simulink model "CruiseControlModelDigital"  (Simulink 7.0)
settings: Solver=ode45  StartTime=0.0  StopTime=100  MaxStep=0.01  RelTol=1e-3
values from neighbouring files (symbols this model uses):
  g = 9.81    [CruiseControlDigital.m]
  m = 1000    [CruiseControlDigital.m]
libraries: cstblocks x10

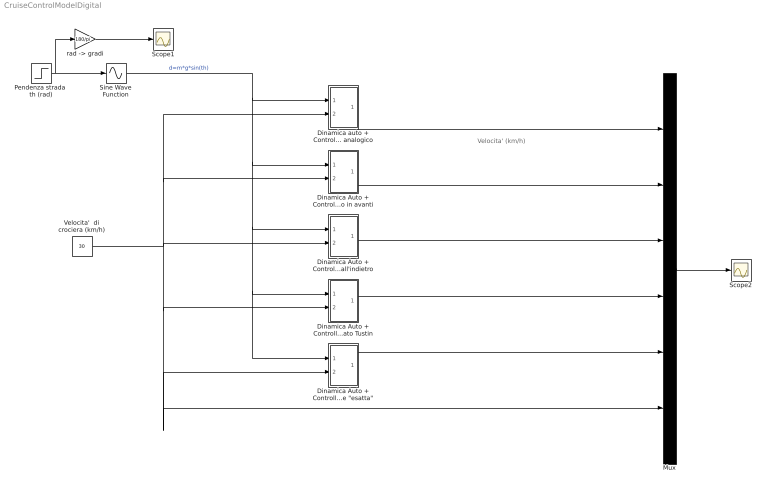
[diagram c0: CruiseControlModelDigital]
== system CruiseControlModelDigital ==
  note: Velocita' (km/h)
  "Dinamica Auto + Controllore digitalizzato Discretizzazione \"esatta\"" : Subsystem
  Dinamica Auto + Controllore digitalizzato Eulero all'indietro : Subsystem
  Dinamica Auto + Controllore digitalizzato Eulero in avanti : Subsystem
  Dinamica Auto + Controllore digitalizzato Tustin : Subsystem
  Dinamica auto + Controllore analogico : Subsystem
  Mux : Mux  Inputs=6
  Pendenza strada  th (rad) : Step  Time=20  After=5*pi/180  SampleTime=0
  Scope1 : Scope
  Scope2 : Scope
  Sine Wave Function : Sin  TimeSource=Use external signal  Amplitude=m*g  SampleTime=0
  Velocita'  di crociera (km/h) : Constant  Value=30  OutDataType=sfix(16)  OutScaling=2^0
  "rad -> gradi" : Gain  Gain=180/pi  ParameterDataType=sfix(16)  ParameterScaling=2^0  OutDataType=sfix(16)  OutScaling=2^0
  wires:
  Pendenza strada  th (rad)/1 -> Sine Wave Function/1, "rad -> gradi"/1
  "rad -> gradi"/1 -> Scope1/1
  Sine Wave Function/1 -> Dinamica auto + Controllore analogico/1(In1), Dinamica Auto + Controllore digitalizzato Eulero in avanti/1(In1), Dinamica Auto + Controllore digitalizzato Eulero all'indietro/1(In1), Dinamica Auto + Controllore digitalizzato Tustin/1(In1), "Dinamica Auto + Controllore digitalizzato Discretizzazione \"esatta\""/1(In1)  "d=m*g*sin(th)"
  Dinamica auto + Controllore analogico/1(Out1) -> Mux/1
  Dinamica Auto + Controllore digitalizzato Eulero in avanti/1(Out1) -> Mux/2
  Dinamica Auto + Controllore digitalizzato Eulero all'indietro/1(Out1) -> Mux/3
  Dinamica Auto + Controllore digitalizzato Tustin/1(Out1) -> Mux/4
  Mux/1 -> Scope2/1
  "Dinamica Auto + Controllore digitalizzato Discretizzazione \"esatta\""/1(Out1) -> Mux/5
  Velocita'  di crociera (km/h)/1 -> Dinamica Auto + Controllore digitalizzato Tustin/2(In2), "Dinamica Auto + Controllore digitalizzato Discretizzazione \"esatta\""/2(In2), Mux/6, Dinamica auto + Controllore analogico/2(In2), Dinamica Auto + Controllore digitalizzato Eulero in avanti/2(In2), Dinamica Auto + Controllore digitalizzato Eulero all'indietro/2(In2)

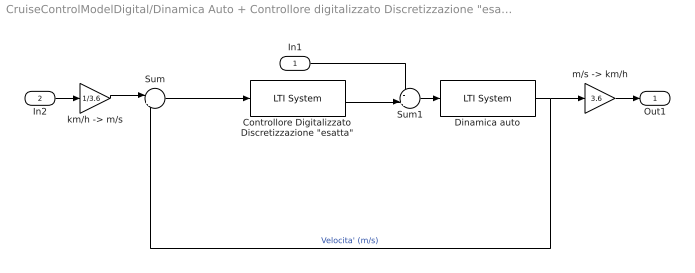
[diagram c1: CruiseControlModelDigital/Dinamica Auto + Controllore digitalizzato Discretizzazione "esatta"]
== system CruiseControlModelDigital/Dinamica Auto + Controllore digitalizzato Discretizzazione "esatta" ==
  In1 : Inport  OutDataType=sfix(16)  OutScaling=2^0
  In2 : Inport  Port=2  OutDataType=sfix(16)  OutScaling=2^0
  "Controllore Digitalizzato Discretizzazione \"esatta\"" : cstblocks/LTI System  SystemSampleTime=-1  sys=Cdz  IC=[]
  Dinamica auto : cstblocks/LTI System  SystemSampleTime=-1  sys=G  IC=[]
  Sum : Sum  Inputs=|+-  OutDataType=sfix(16)  OutScaling=2^0
  Sum1 : Sum  Inputs=-+|  OutDataType=sfix(16)  OutScaling=2^0
  "km/h -> m/s" : Gain  Gain=1/3.6  ParameterDataType=sfix(16)  ParameterScaling=2^0  OutDataType=sfix(16)  OutScaling=2^0
  "m/s -> km/h" : Gain  Gain=3.6  ParameterDataType=sfix(16)  ParameterScaling=2^0  OutDataType=sfix(16)  OutScaling=2^0
  Out1 : Outport  OutDataType=sfix(16)  OutScaling=2^0
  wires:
  "km/h -> m/s"/1 -> Sum/1
  "Controllore Digitalizzato Discretizzazione \"esatta\""/1 -> Sum1/2
  Sum1/1 -> Dinamica auto/1
  Dinamica auto/1 -> "m/s -> km/h"/1, Sum/2  "Velocita' (m/s)"
  Sum/1 -> "Controllore Digitalizzato Discretizzazione \"esatta\""/1
  In1/1 -> Sum1/1
  In2/1 -> "km/h -> m/s"/1
  "m/s -> km/h"/1 -> Out1/1

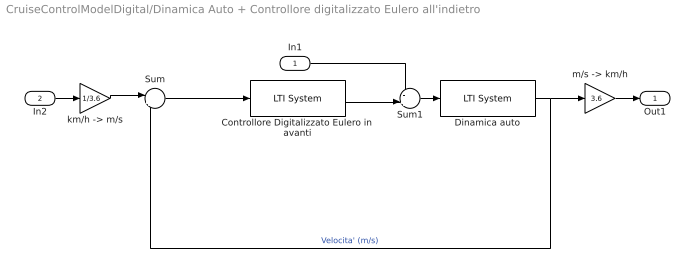
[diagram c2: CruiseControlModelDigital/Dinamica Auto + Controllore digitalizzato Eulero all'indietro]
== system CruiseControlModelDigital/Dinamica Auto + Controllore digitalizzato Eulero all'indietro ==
  In1 : Inport  OutDataType=sfix(16)  OutScaling=2^0
  In2 : Inport  Port=2  OutDataType=sfix(16)  OutScaling=2^0
  Controllore Digitalizzato Eulero in avanti : cstblocks/LTI System  SystemSampleTime=-1  sys=Cdb  IC=[]
  Dinamica auto : cstblocks/LTI System  SystemSampleTime=-1  sys=G  IC=[]
  Sum : Sum  Inputs=|+-  OutDataType=sfix(16)  OutScaling=2^0
  Sum1 : Sum  Inputs=-+|  OutDataType=sfix(16)  OutScaling=2^0
  "km/h -> m/s" : Gain  Gain=1/3.6  ParameterDataType=sfix(16)  ParameterScaling=2^0  OutDataType=sfix(16)  OutScaling=2^0
  "m/s -> km/h" : Gain  Gain=3.6  ParameterDataType=sfix(16)  ParameterScaling=2^0  OutDataType=sfix(16)  OutScaling=2^0
  Out1 : Outport  OutDataType=sfix(16)  OutScaling=2^0
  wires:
  "km/h -> m/s"/1 -> Sum/1
  Controllore Digitalizzato Eulero in avanti/1 -> Sum1/2
  Sum1/1 -> Dinamica auto/1
  Dinamica auto/1 -> "m/s -> km/h"/1, Sum/2  "Velocita' (m/s)"
  Sum/1 -> Controllore Digitalizzato Eulero in avanti/1
  In1/1 -> Sum1/1
  In2/1 -> "km/h -> m/s"/1
  "m/s -> km/h"/1 -> Out1/1

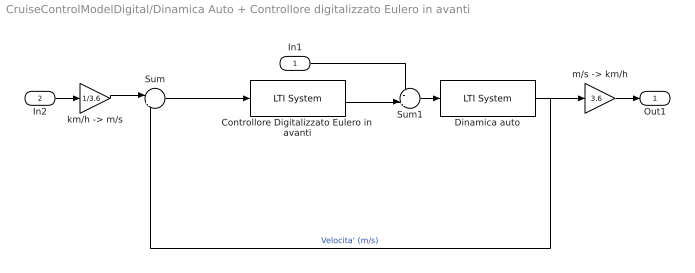
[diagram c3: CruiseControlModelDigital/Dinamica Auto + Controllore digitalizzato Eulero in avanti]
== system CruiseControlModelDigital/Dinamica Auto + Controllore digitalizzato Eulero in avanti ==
  In1 : Inport  OutDataType=sfix(16)  OutScaling=2^0
  In2 : Inport  Port=2  OutDataType=sfix(16)  OutScaling=2^0
  Controllore Digitalizzato Eulero in avanti : cstblocks/LTI System  SystemSampleTime=-1  sys=Cdf  IC=[]
  Dinamica auto : cstblocks/LTI System  SystemSampleTime=-1  sys=G  IC=[]
  Sum : Sum  Inputs=|+-  OutDataType=sfix(16)  OutScaling=2^0
  Sum1 : Sum  Inputs=-+|  OutDataType=sfix(16)  OutScaling=2^0
  "km/h -> m/s" : Gain  Gain=1/3.6  ParameterDataType=sfix(16)  ParameterScaling=2^0  OutDataType=sfix(16)  OutScaling=2^0
  "m/s -> km/h" : Gain  Gain=3.6  ParameterDataType=sfix(16)  ParameterScaling=2^0  OutDataType=sfix(16)  OutScaling=2^0
  Out1 : Outport  OutDataType=sfix(16)  OutScaling=2^0
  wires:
  "km/h -> m/s"/1 -> Sum/1
  Controllore Digitalizzato Eulero in avanti/1 -> Sum1/2
  Sum1/1 -> Dinamica auto/1
  Dinamica auto/1 -> "m/s -> km/h"/1, Sum/2  "Velocita' (m/s)"
  Sum/1 -> Controllore Digitalizzato Eulero in avanti/1
  In1/1 -> Sum1/1
  In2/1 -> "km/h -> m/s"/1
  "m/s -> km/h"/1 -> Out1/1

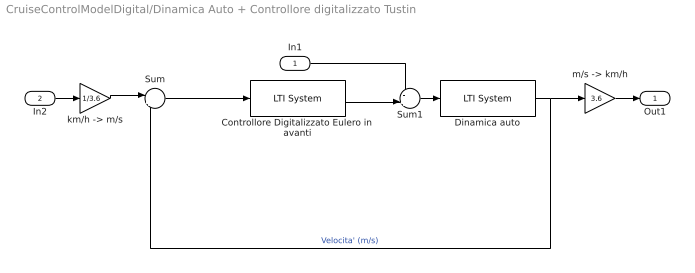
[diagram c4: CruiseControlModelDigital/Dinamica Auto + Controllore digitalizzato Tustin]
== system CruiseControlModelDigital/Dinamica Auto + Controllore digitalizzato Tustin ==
  In1 : Inport  OutDataType=sfix(16)  OutScaling=2^0
  In2 : Inport  Port=2  OutDataType=sfix(16)  OutScaling=2^0
  Controllore Digitalizzato Eulero in avanti : cstblocks/LTI System  SystemSampleTime=-1  sys=Cdt  IC=[]
  Dinamica auto : cstblocks/LTI System  SystemSampleTime=-1  sys=G  IC=[]
  Sum : Sum  Inputs=|+-  OutDataType=sfix(16)  OutScaling=2^0
  Sum1 : Sum  Inputs=-+|  OutDataType=sfix(16)  OutScaling=2^0
  "km/h -> m/s" : Gain  Gain=1/3.6  ParameterDataType=sfix(16)  ParameterScaling=2^0  OutDataType=sfix(16)  OutScaling=2^0
  "m/s -> km/h" : Gain  Gain=3.6  ParameterDataType=sfix(16)  ParameterScaling=2^0  OutDataType=sfix(16)  OutScaling=2^0
  Out1 : Outport  OutDataType=sfix(16)  OutScaling=2^0
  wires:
  "km/h -> m/s"/1 -> Sum/1
  Controllore Digitalizzato Eulero in avanti/1 -> Sum1/2
  Sum1/1 -> Dinamica auto/1
  Dinamica auto/1 -> "m/s -> km/h"/1, Sum/2  "Velocita' (m/s)"
  Sum/1 -> Controllore Digitalizzato Eulero in avanti/1
  In1/1 -> Sum1/1
  In2/1 -> "km/h -> m/s"/1
  "m/s -> km/h"/1 -> Out1/1

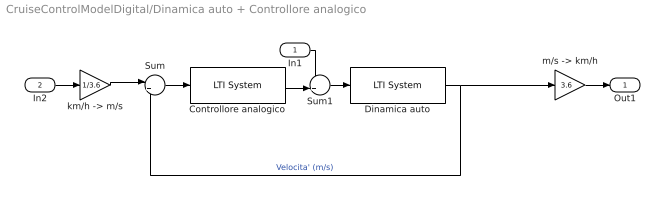
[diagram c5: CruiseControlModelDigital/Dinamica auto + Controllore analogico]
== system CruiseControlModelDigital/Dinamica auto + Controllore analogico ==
  In1 : Inport  OutDataType=sfix(16)  OutScaling=2^0
  In2 : Inport  Port=2  OutDataType=sfix(16)  OutScaling=2^0
  Controllore analogico : cstblocks/LTI System  SystemSampleTime=-1  sys=C  IC=[]
  Dinamica auto : cstblocks/LTI System  SystemSampleTime=-1  sys=G  IC=[]
  Sum : Sum  Inputs=|+-  OutDataType=sfix(16)  OutScaling=2^0
  Sum1 : Sum  Inputs=-+|  OutDataType=sfix(16)  OutScaling=2^0
  "km/h -> m/s" : Gain  Gain=1/3.6  ParameterDataType=sfix(16)  ParameterScaling=2^0  OutDataType=sfix(16)  OutScaling=2^0
  "m/s -> km/h" : Gain  Gain=3.6  ParameterDataType=sfix(16)  ParameterScaling=2^0  OutDataType=sfix(16)  OutScaling=2^0
  Out1 : Outport  OutDataType=sfix(16)  OutScaling=2^0
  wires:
  "km/h -> m/s"/1 -> Sum/1
  Controllore analogico/1 -> Sum1/2
  Sum1/1 -> Dinamica auto/1
  Dinamica auto/1 -> Sum/2, "m/s -> km/h"/1  "Velocita' (m/s)"
  Sum/1 -> Controllore analogico/1
  In1/1 -> Sum1/1
  In2/1 -> "km/h -> m/s"/1
  "m/s -> km/h"/1 -> Out1/1
